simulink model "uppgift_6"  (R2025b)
settings: Solver=VariableStepAuto  StartTime=0.0  StopTime=10.0  RelTol=1e-3
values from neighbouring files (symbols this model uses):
  AFs = 14.6    [Lektion_2.m]
  Ki = 0.1    [Lektion_2.m]
  Kp = 0    [Lektion_2.m]

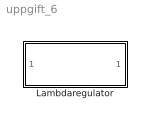
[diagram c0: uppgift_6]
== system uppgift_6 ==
  Lambdaregulator : Subsystem

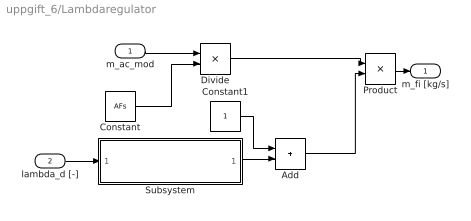
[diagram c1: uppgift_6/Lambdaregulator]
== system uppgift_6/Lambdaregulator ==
  m_ac_mod : Inport
  lambda_d [-] : Inport  Port=2
  Add : Sum
  Constant : Constant  Value=AFs
  Constant1 : Constant
  Divide : Product  Inputs=*/
  Product : Product
  Subsystem : Subsystem
  m_fi [kg/s] : Outport
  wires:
  m_ac_mod/1 -> Divide/1
  Constant/1 -> Divide/2
  Constant1/1 -> Add/1
  Divide/1 -> Product/1
  Add/1 -> Product/2
  Product/1 -> m_fi [kg/s]/1
  Subsystem/1("Lambda_controlled ") -> Add/2
  lambda_d [-]/1 -> Subsystem/1(lambda_d)

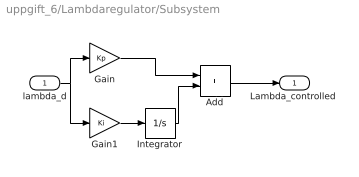
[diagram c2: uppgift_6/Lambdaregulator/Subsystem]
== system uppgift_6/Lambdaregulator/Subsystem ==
  lambda_d : Inport
  Add : Sum
  Gain : Gain  Gain=Kp
  Gain1 : Gain  Gain=Ki
  Integrator : Integrator
  "Lambda_controlled " : Outport
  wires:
  Add/1 -> "Lambda_controlled "/1
  Gain1/1 -> Integrator/1
  Integrator/1 -> Add/2
  lambda_d/1 -> Gain/1, Gain1/1
  Gain/1 -> Add/1
